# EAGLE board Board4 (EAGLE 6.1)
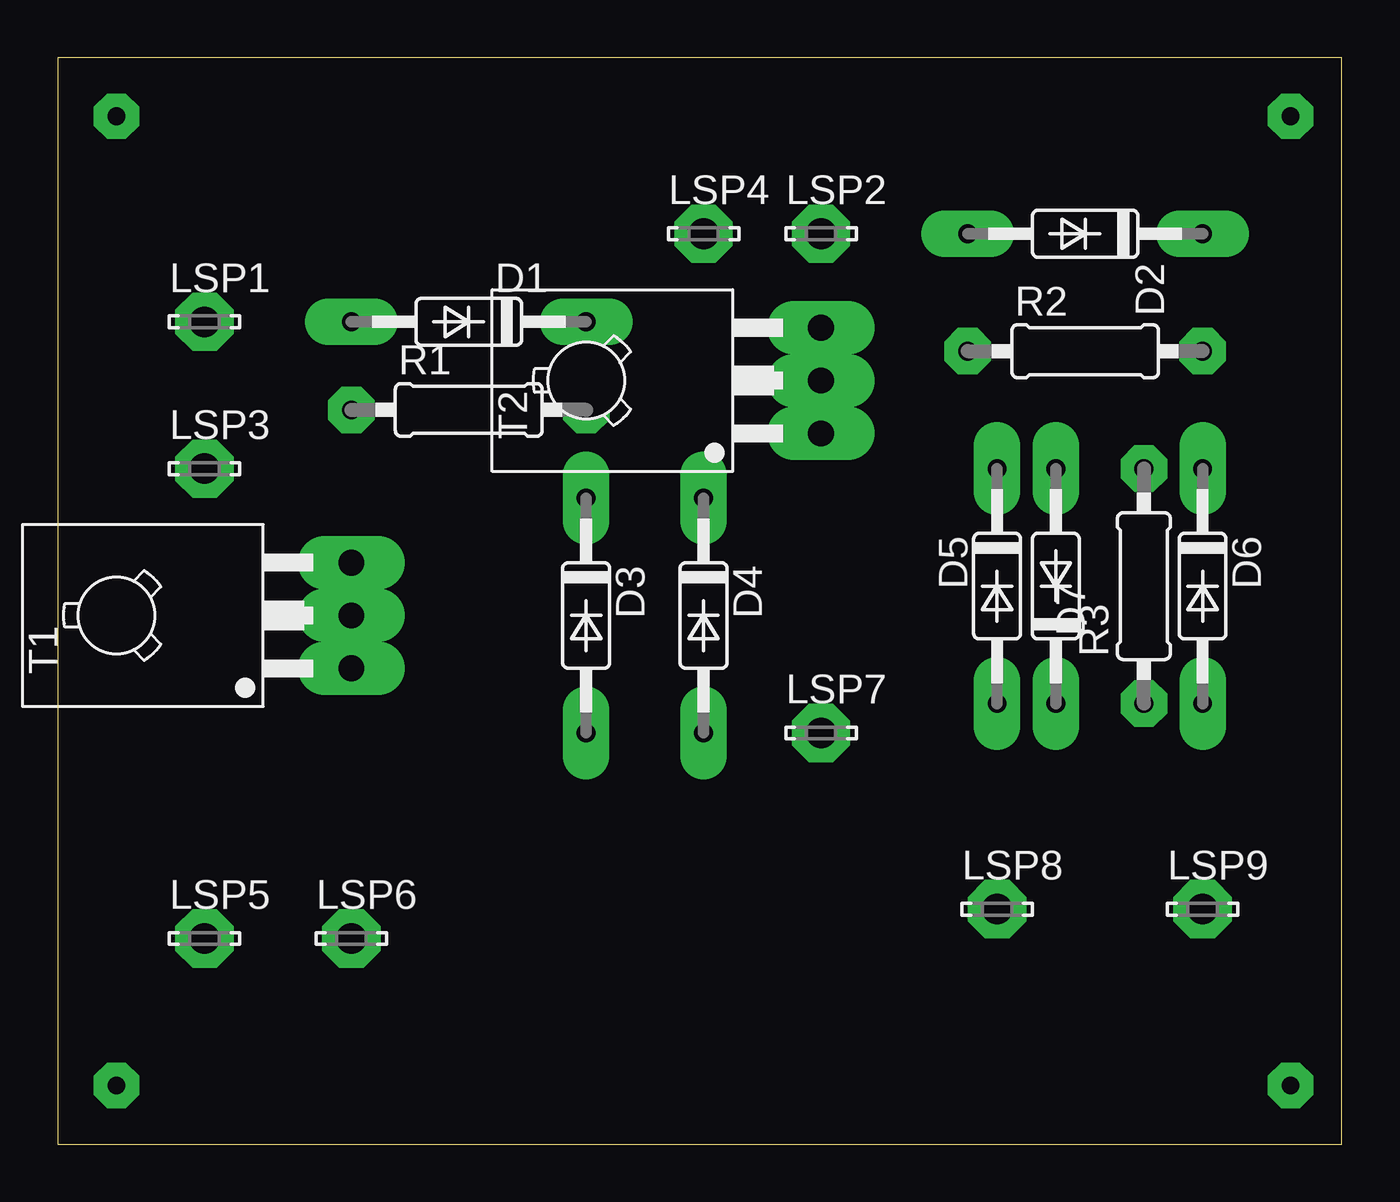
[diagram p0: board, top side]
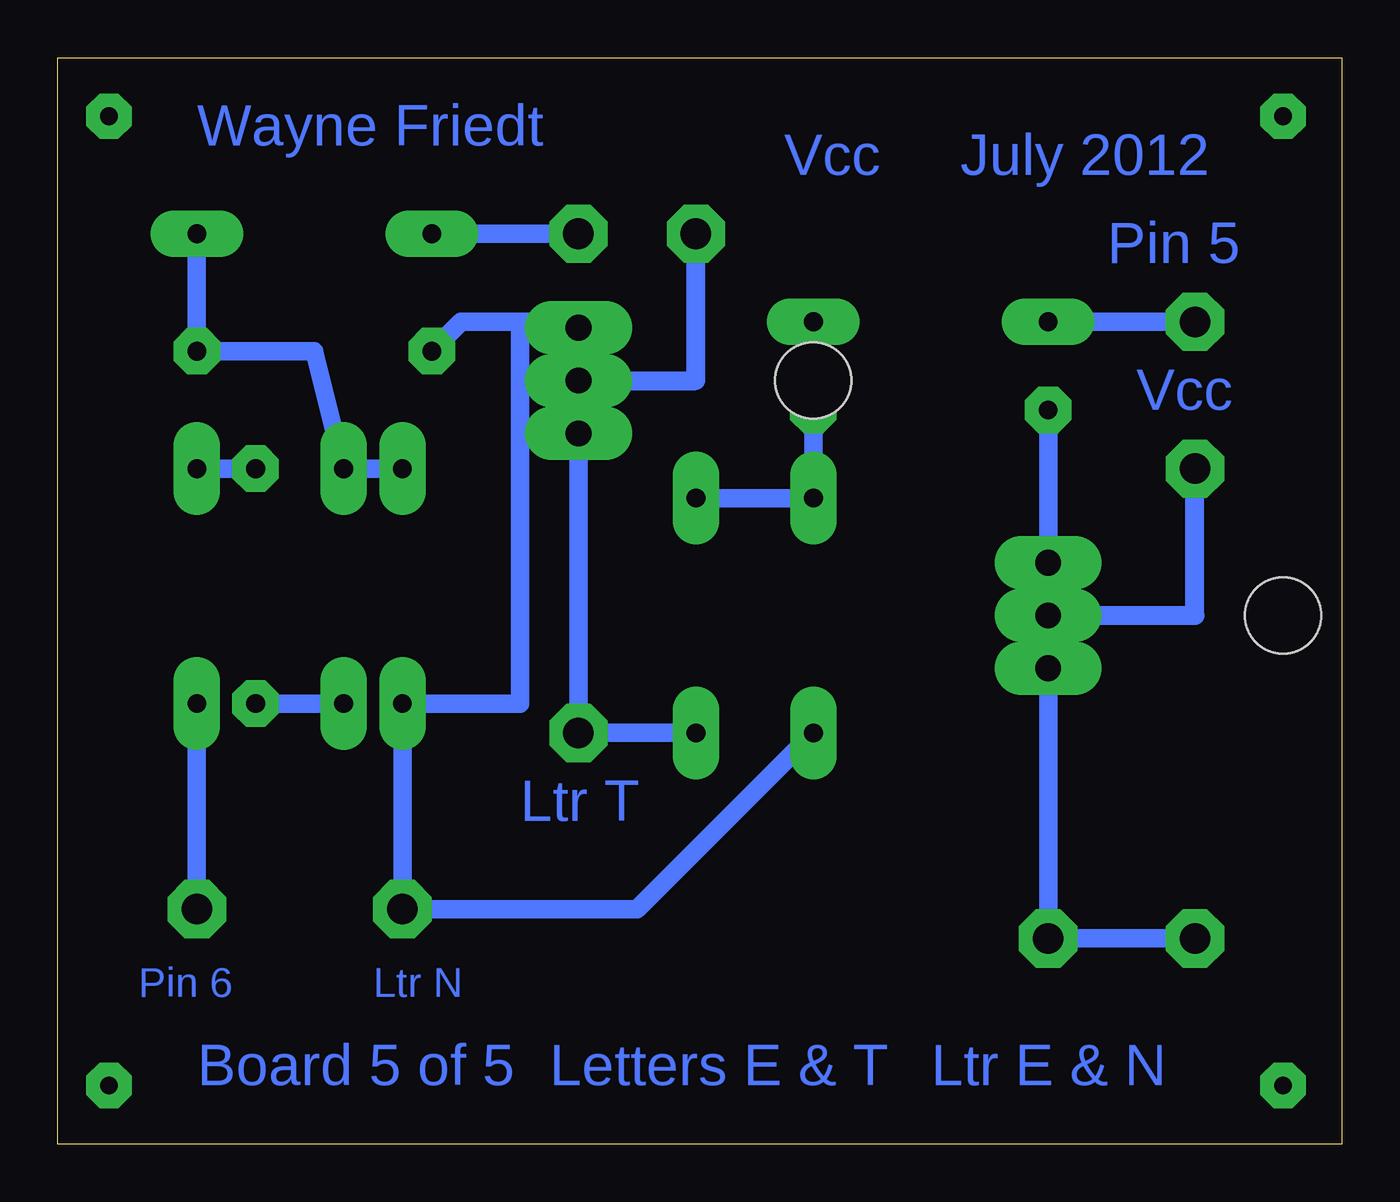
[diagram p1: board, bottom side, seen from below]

Size 55.55 x 46.98 mm. Coordinates in mm from the lower left corner, seen from the top.
Outline: 0,0 55.55,0 55.55,46.98 0,46.98 0,0
Copper layers (1*16): Top 0.035mm / dielectric 1.5mm / Bottom 0.035mm
Design rules: minimum track width 0.8mm, minimum drill 0.8mm, track to track 0.8mm, track to pad 0.8mm, pad to pad 0.45mm, via to via 0.8mm, smd to smd 8mil, copper to edge 10mil, drill to drill 8mil, minimum pad ring 0.6mm, minimum via ring 0.6mm, stop-mask expansion 0mil, vias tented up to drill 0mil, thermal gap 10mil

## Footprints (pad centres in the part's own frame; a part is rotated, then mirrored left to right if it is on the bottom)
DO35-10 = drill 0.813 long: A 5.08,0; C -5.08,0
LSP13 = drill 1.321 pad 2.159 octagon: MP 0,0
0207/10 = drill 0.813 octagon: 1 -5.08,0; 2 5.08,0
TO126 = drill 1.118 long: 1 -2.286,-5.08; 2 0,-5.08; 3 2.286,-5.08 | hole 3.302: 0,5.08

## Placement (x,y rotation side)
D1  1N4148DO35-10  [DO35-10]  17.78,35.56 180 top
D2  1N4148DO35-10  [DO35-10]  44.45,39.37 180 top
D3  1N4148DO35-10  [DO35-10]  22.86,22.86 270 top
D4  1N4148DO35-10  [DO35-10]  27.94,22.86 270 top
D5  1N4148DO35-10  [DO35-10]  40.64,24.13 270 top
D6  1N4148DO35-10  [DO35-10]  49.53,24.13 270 top
D7  1N4148DO35-10  [DO35-10]  43.18,24.13 90 top
LSP1  LSP13  [LSP13]  6.35,35.56 0 top
LSP2  LSP13  [LSP13]  33.02,39.37 0 top
LSP3  LSP13  [LSP13]  6.35,29.21 0 top
LSP4  LSP13  [LSP13]  27.94,39.37 0 top
LSP5  LSP13  [LSP13]  6.35,8.89 0 top
LSP6  LSP13  [LSP13]  12.7,8.89 0 top
LSP7  LSP13  [LSP13]  33.02,17.78 0 top
LSP8  LSP13  [LSP13]  40.64,10.16 0 top
LSP9  LSP13  [LSP13]  49.53,10.16 0 top
R1  [0207/10]  17.78,31.75 0 top
R2  [0207/10]  44.45,34.29 0 top
R3  330R  [0207/10]  46.99,24.13 90 top
T1  BD139  [TO126]  7.62,22.86 90 top
T2  BD139  [TO126]  27.94,33.02 90 top

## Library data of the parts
D1-D7 = diode
LSP1-LSP9 = solpad
R1-R3 = resistor
T1 T2 = transistor

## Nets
N$1: R1.1 T1.3
N$2: D1.C D3.C D4.C R1.2
N$3: D1.A LSP1.MP
N$4: LSP3.MP T1.2
N$5: D2.A LSP2.MP
N$6: D2.C D5.C D7.A R2.2
N$7: D3.A D5.A LSP8.MP R2.1 T2.3
N$8: LSP4.MP T2.2
N$9: D4.A LSP7.MP T2.1
N$10: D7.C R3.1
N$11: LSP5.MP LSP6.MP T1.1
N$12: D6.C R3.2
N$13: D6.A LSP9.MP

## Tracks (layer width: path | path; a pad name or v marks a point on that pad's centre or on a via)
N$1
  Bottom 0.8: T1.3 R1.1
N$2
  Bottom 0.8: D4.C D3.C R1.2 D1.C
N$3
  Bottom 0.8: LSP1.MP D1.A
N$4
  Bottom 0.813: T1.2 6.35,22.86 LSP3.MP
N$5
  Bottom 0.8: LSP2.MP D2.A
N$6
  Bottom 0.8: D2.C R2.2 44.45,34.29 D7.A D5.C
N$7
  Bottom 0.8: D3.A 30.48,10.16 LSP8.MP D5.A 35.56,19.05 35.56,35.56 | R2.1 38.1,35.56 35.56,35.56 | 35.56,35.56 33.02,35.56 T2.3
N$8
  Bottom 0.813: T2.2 27.94,33.02 LSP4.MP
N$9
  Bottom 0.8: D4.A LSP7.MP T2.1
N$10
  Bottom 0.8: R3.1 D7.C
N$11
  Bottom 0.8: T1.1 LSP6.MP LSP5.MP
N$12
  Bottom 0.8: D6.C R3.2
N$13
  Bottom 0.8: LSP9.MP D6.A
S$1  (via drill 0.76)
  other vias: 2.54,2.54 2.54,44.45 53.34,44.45 53.34,2.54

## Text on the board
Bottom: Wayne Friedt | July 2012 | Vcc | Pin 5 | Vcc | Ltr T | Ltr N | Pin 6 | Ltr E & N | Letters E & T | Board 5 of 5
